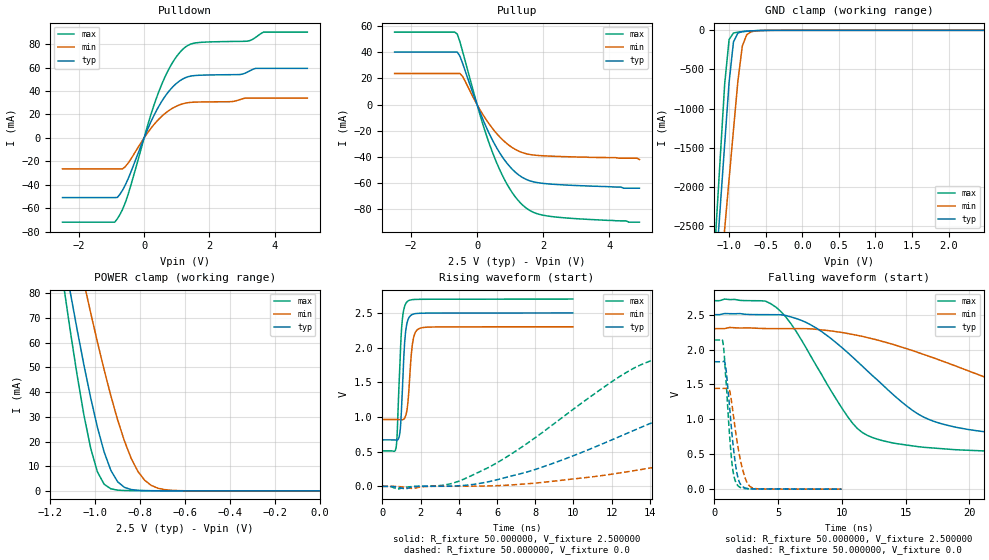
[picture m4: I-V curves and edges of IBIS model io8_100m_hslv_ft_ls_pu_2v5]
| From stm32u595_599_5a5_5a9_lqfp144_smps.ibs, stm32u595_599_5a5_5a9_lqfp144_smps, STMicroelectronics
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|   Model io8_100m_hslv_ft_ls_pu_2v5
[Model]  io8_100m_hslv_ft_ls_pu_2v5
Model_type I/O
Polarity   Non-Inverting
Enable   Active-Low
Vinl =   0.750000V
Vinh =   1.750000V
Vmeas =  1.250000V
Cref =   50.000000pF
Rref =   100.000000M
Vref =   0.0V
C_comp   3.340800pF   3.338500pF   3.380300pF
[Temperature Range]   25.000000   0.140000k   -40.000000
[Pullup Reference]   2.500000V   2.300000V   2.700000V
[Pulldown Reference]   0.0V   0.0V   0.0V
[POWER Clamp Reference]   2.500000V   2.300000V   2.700000V
[GND Clamp Reference]   0.0V   0.0V   0.0V
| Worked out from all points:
|   slope of the pulldown table from 0 to 0.375 V, typ, clamps not added: 16.1 ohm
|   slope of the pullup table from 0 to 0.375 V, typ, clamps not added: 16.6 ohm
|   GND clamp passes 1 mA (typ) near -0.50 V on its own axis
|   POWER clamp passes 1 mA (typ) near -0.85 V on its own axis
|   rising waveform, R_fixture 50.000000, V_fixture 2.500000: 20-80 % time 197ps typ, 222ps min, 201ps max; typ from 0.671 V to 2.5 V
|   rising waveform, R_fixture 50.000000, V_fixture 0.0: 20-80 % time 10ns typ, 18.1ns min, 6.68ns max; typ from 0.001 V to 1.83 V
|   falling waveform, R_fixture 50.000000, V_fixture 2.500000: 20-80 % time 7.08ns typ, 14.2ns min, 4.42ns max; typ from 2.5 V to 0.671 V
|   falling waveform, R_fixture 50.000000, V_fixture 0.0: 20-80 % time 601ps typ, 785ps min, 497ps max; typ from 1.83 V to 0.001 V
[Pulldown]
|Voltage   I(typ)   I(min)   I(max)
-2.5V     -51mA      -26.45mA   -72.04mA
-900mV    -51mA      -26.45mA   -72.04mA
-820mV    -50.89mA   -26.45mA   -69.09mA
-500mV    -35.59mA   -21.93mA   -49.09mA
140mV     9.488mA    5.639mA    13.76mA
460mV     27.5mA     16.24mA    40.22mA
860mV     43.07mA    25.18mA    63.88mA
1.26V     51.38mA    29.65mA    77.49mA
1.66V     53.45mA    30.63mA    81.42mA
3.18V     56.44mA    33.99mA    82.68mA
3.66V     59.4mA     33.99mA    90.38mA
5V        59.4mA     33.99mA    90.38mA
[Pullup]
|Voltage   I(typ)   I(min)   I(max)
-2.5V     40.22mA    23.82mA    55.51mA
-680mV    40.22mA    23.82mA    55.51mA
-600mV    40.22mA    23.82mA    53.96mA
-440mV    31.7mA     21.6mA     40.82mA
120mV     -7.857mA   -5.279mA   -10.51mA
520mV     -29.75mA   -19.94mA   -40.02mA
760mV     -39.82mA   -26.61mA   -53.83mA
1V        -47.69mA   -31.74mA   -64.85mA
1.48V     -57.16mA   -37.55mA   -79.04mA
1.8V      -59.59mA   -38.81mA   -83.34mA
2.28V     -60.93mA   -39.5mA    -85.75mA
4.92V     -64mA      -42mA      -90mA
[GND_clamp]
|Voltage   I(typ)   I(min)   I(max)
-2.5V     -9.446A    -9.524A    -9.146A
-1.18V    -3.045A    -3.8A      -2.552A
-1.12V    -2.248A    -3.166A    -1.614A
-1.06V    -1.452A    -2.533A    -685.3mA
-1V       -665mA     -1.901A    -117.9mA
-940mV    -148mA     -1.272A    -34.32mA
-880mV    -35.13mA   -651.5mA   -22.79mA
-820mV    -16mA      -203.9mA   -17.07mA
-760mV    -10.46mA   -56.88mA   -12.26mA
-700mV    -7.068mA   -18.52mA   -8.146mA
-400mV    -103.3uA   -375.9uA   -42.12uA
2.48V     0A         14.84nA    0A
[POWER_clamp]
|Voltage   I(typ)   I(min)   I(max)
-2.49V    881.1mA    773.1mA    1.07A
-1.14V    95.32mA    122.8mA    82.93mA
-1.11V    79.97mA    109.7mA    64.26mA
-1.05V    50.95mA    84.3mA     30.69mA
-1.02V    37.7mA     72.08mA    17.29mA
-990mV    25.79mA    60.29mA    7.738mA
-930mV    8.312mA    38.47mA    853.6uA
-900mV    3.712mA    28.81mA    314.2uA
-840mV    566.7uA    13.29mA    124.4uA
-780mV    119.5uA    4.365mA    94.68uA
-660mV    39.4uA     251.7uA    58.31uA
0V        0A         18.89nA    0A
[Ramp]
| variable   typ   min   max
dV/dt_r  1.09488/9.98551n   0.86563/18.06231n   1.28167/6.66974n
dV/dt_f  1.09764/7.06759n   0.80159/14.14468n   1.31314/4.41540n
R_load = 50.000000
[Rising Waveform]
R_fixture= 50.000000
V_fixture= 2.500000
V_fixture_min= 2.300000
V_fixture_max= 2.700000
|time   V(typ)   V(min)   V(max)
0s        670.6mV    964mV      511.4mV
720.7ps   666.9mV    964mV      564.3mV
780.8ps   668.5mV    963.9mV    794mV
920.9ps   782.2mV    962.8mV    1.773V
1.021ns   1.228V     960.3mV    2.33V
1.161ns   2.052V     982mV      2.591V
1.321ns   2.386V     1.17V      2.668V
1.582ns   2.48V      2.064V     2.692V
1.922ns   2.495V     2.273V     2.696V
9.97ns    2.5V       2.3V       2.7V
[Rising Waveform]
R_fixture= 50.000000
V_fixture= 0.0
V_fixture_min= 0.0
V_fixture_max= 0.0
|time   V(typ)   V(min)   V(max)
0s        693.1uV    785.1uV    681.4uV
2.803ns   1.835mV    1.339mV    6.352mV
4.404ns   17.06mV    2.481mV    121.5mV
8.008ns   244.6mV    47.18mV    703.3mV
14.01ns   906.6mV    264.8mV    1.807V
18.82ns   1.425V     504.5mV    2.034V
21.62ns   1.596V     652mV      2.082V
33.23ns   1.786V     1.175V     2.131V
50.05ns   1.822V     1.388V     2.137V
199.4ns   1.825V     1.444V     2.137V
[Falling Waveform]
R_fixture= 50.000000
V_fixture= 2.500000
V_fixture_min= 2.300000
V_fixture_max= 2.700000
|time   V(typ)   V(min)   V(max)
0s        2.5V       2.3V       2.7V
4.004ns   2.5V       2.301V     2.694V
5.205ns   2.499V     2.3V       2.547V
8.008ns   2.306V     2.29V      1.766V
11.61ns   1.762V     2.189V     811.6mV
15.62ns   1.121V     1.982V     619mV
18.82ns   893mV      1.772V     567.1mV
29.23ns   725.1mV    1.222V     521.5mV
49.25ns   677.4mV    1.019V     512mV
199.4ns   670.6mV    964mV      511.4mV
[Falling Waveform]
R_fixture= 50.000000
V_fixture= 0.0
V_fixture_min= 0.0
V_fixture_max= 0.0
|time   V(typ)   V(min)   V(max)
0s        1.825V     1.444V     2.137V
620.6ps   1.825V     1.444V     2.139V
840.8ps   1.798V     1.444V     1.73V
1.141ns   1.277V     1.439V     892.3mV
1.361ns   819.3mV    1.23V      399.7mV
1.562ns   481.3mV    955.9mV    165mV
1.822ns   183.9mV    631mV      55.15mV
2.362ns   21.34mV    187.4mV    9.724mV
2.943ns   4.876mV    22.97mV    5.281mV
9.97ns    693.1uV    785.1uV    681.4uV
